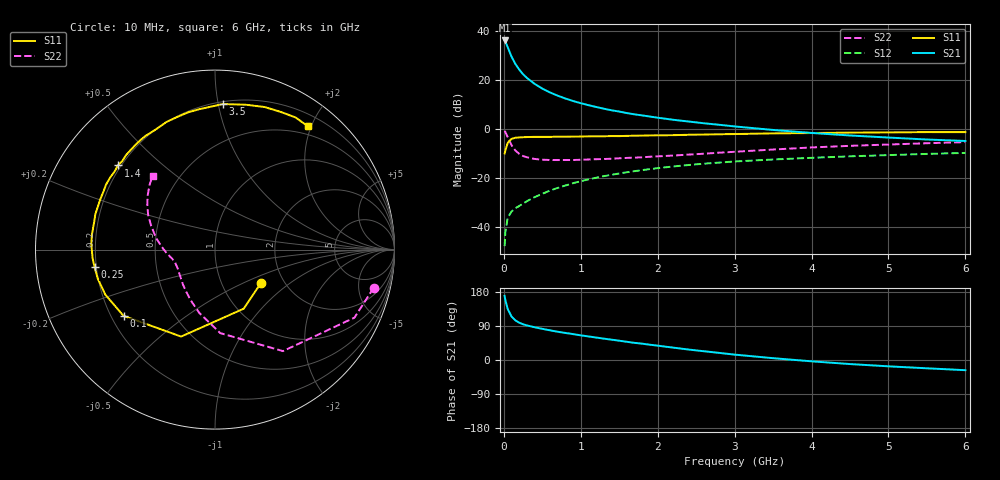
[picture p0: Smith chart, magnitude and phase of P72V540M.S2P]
! SIEMENS Small Signal Semiconductors
! BFP196
! Si NPN RF Bipolar Junction Transistor in SOT143
! VCE = 2.5 V  IC = 40 mA
! Common Emitter S-Parameters:  May  1996
# GHz  S  MA  R  50
!  f  S11  S21  S12  S22
! GHz  MAG  ANG  MAG  ANG  MAG  ANG  MAG  ANG
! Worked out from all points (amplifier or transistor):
!   36 points, 10 MHz to 6 GHz, reference 50 ohm
!   highest |S21| = 36.0 dB at 10 MHz (marker M1)
!   |S21| within 3 dB of that: start of sweep to 53.84 MHz
!   unconditionally stable (mu >= 1): 476.8 MHz to 4.284 GHz
!   at 250 MHz: K = 0.81, MSG = 26.3 dB, |S12| = -30.4 dB
!   at 1.4 GHz: K = 1.09, MAG = 11.3 dB, |S12| = -18.7 dB
!   at 6 GHz: K = 0.99, MSG = 2.4 dB, |S12| = -9.8 dB
!   S11 on the Smith chart (normalised r, x): 10 MHz: 1.52, -0.64; 100 MHz: 0.25, -0.31; 250 MHz: 0.19, -0.07; 1.4 GHz: 0.19, +0.36; 3.5 GHz: 0.22, +1.03; 6 GHz: 0.37, +1.95
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0.01  0.3166 -36.4  63.38 169.2  0.0041 82.0  0.9094 -13.5
0.02  0.366 -64.1  59.89 157.9  0.0079 70.3  0.8645 -26.0
0.05  0.52 -111.3  46.44 134.7  0.0155 55.6  0.6807 -56.2
0.1  0.6292 -144.1  29.7 114.6  0.0208 47.4  0.4661 -86.4
0.15  0.6607 -157.7  21.04 104.5  0.0243 46.4  0.3631 -104.0
0.2  0.6729 -166.1  16.19 98.5  0.027 48.9  0.3112 -116.2
0.25  0.678 -171.7  12.99 94.3  0.0302 51.5  0.2808 -125.6
0.3  0.6837 -176.0  10.93 91.2  0.0338 53.3  0.265 -132.1
0.4  0.6901 177.2  8.287 86.4  0.0409 57.1  0.2449 -142.1
0.5  0.6905 172.5  6.627 82.3  0.0477 58.9  0.2365 -148.7
0.6  0.6901 167.8  5.534 78.3  0.0557 60.1  0.233 -153.1
0.7  0.6953 163.6  4.761 74.5  0.063 60.8  0.2325 -156.5
0.9  0.6978 156.3  3.707 68.3  0.0786 60.3  0.2333 -161.8
1.1  0.707 149.1  3.05 62.1  0.0939 59.0  0.2387 -165.2
1.4  0.7159 139.1  2.4 53.7  0.1164 55.9  0.2473 -169.3
1.7  0.7276 129.9  1.981 45.2  0.1381 52.0  0.2606 -173.9
2.2  0.7463 116.2  1.539 32.7  0.1718 45.1  0.287 179.5
2.8  0.7792 101.1  1.215 18.8  0.2066 36.6  0.3287 170.0
3.5  0.8123 86.9  0.954 4.8  0.2389 26.8  0.381 159.3
4.5  0.8413 70.7  0.736 -10.7  0.277 15.0  0.453 146.4
5.5  0.8623 58.6  0.609 -21.9  0.3102 4.2  0.512 135.5
6  0.8603 52.9  0.569 -26.9  0.3252 -1.6  0.5391 130.2
